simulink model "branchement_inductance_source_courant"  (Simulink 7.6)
settings: Solver=ode15s  StartTime=0.0  StopTime=0.015  RelTol=1e-3
StopFcn:
  | close all
  | load VI.mat
  | plotyy(x(1,:),x(2,:),x(1,:),x(3,:))
  | grid
  | title('Tension et courant dans le circuit LC')
  | xlabel('temps')
libraries: powerlib x8

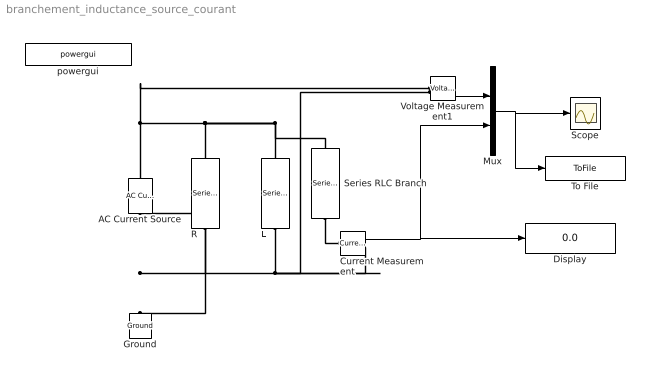
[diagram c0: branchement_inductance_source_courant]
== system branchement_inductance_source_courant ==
  AC Current Source : powerlib/Electrical Sources/AC Current Source  DialogController=POWERSYS.PowerSysDialog  SystemSampleTime=-1  Amplitude=10  Phase=0  Frequency=60  SampleTime=0  Measurements=None
  Current Measurement : powerlib/Measurements/Current Measurement  DialogController=POWERSYS.PowerSysDialog  SystemSampleTime=-1  PhasorSimulation=off  OutputType=Complex  PSBequivalent=0
  Display : Display
  Ground : powerlib/Elements/Ground  DialogController=POWERSYS.PowerSysDialog  PhysicalDomain=powersysdomain  SubClassName=unknown  LeftPortType=p1  RightPortType=p1  LConnTagsString=a
  L : powerlib/Elements/Series RLC Branch  DialogController=POWERSYS.PowerSysDialog  PhysicalDomain=powersysdomain  SubClassName=unknown  LeftPortType=p1  RightPortType=p1  LConnTagsString=__new0  RConnTagsString=__new0  BranchType=L  Resistance=1  Inductance=1e-3  SetiL0=off  InitialCurrent=0  Capacitance=1e-6  Setx0=off  InitialVoltage=0  Measurements=None
  Mux : Mux  Inputs=2
  R : powerlib/Elements/Series RLC Branch  DialogController=POWERSYS.PowerSysDialog  PhysicalDomain=powersysdomain  SubClassName=unknown  LeftPortType=p1  RightPortType=p1  LConnTagsString=__new0  RConnTagsString=__new0  BranchType=R  Resistance=1e6  Inductance=1e-3  SetiL0=off  InitialCurrent=0  Capacitance=1e-6  Setx0=off  InitialVoltage=0  Measurements=None
  Scope : Scope
  Series RLC Branch : powerlib/Elements/Series RLC Branch  DialogController=POWERSYS.PowerSysDialog  PhysicalDomain=powersysdomain  SubClassName=unknown  LeftPortType=p1  RightPortType=p1  LConnTagsString=__new0  RConnTagsString=__new0  BranchType=RL  Resistance=1  Inductance=1e-3  SetiL0=off  InitialCurrent=0  Capacitance=1e-6  Setx0=off  InitialVoltage=0  Measurements=None
  To File : ToFile  Filename=VI.mat  MatrixName=x
  Voltage Measurement1 : powerlib/Measurements/Voltage Measurement  DialogController=POWERSYS.PowerSysDialog  SystemSampleTime=-1  PhasorSimulation=off  OutputType=Complex  PSBequivalent=0
  powergui : powerlib/powergui  Priority=1  SystemSampleTime=-1  SimulationMode=Continuous  SampleTime=50e-6  frequency=60  SPID=off  DisableSnubberDevices=off  DisableRonSwitches=off  DisableVfSwitches=off  SwTol=0  Interpol=off  frequencyindice=60  echomessages=off  HookPort=off  DisplayEquations=off  FunctionMessages=off  EnableUseOfTLC=off  x0status=blocks  RestoreLinks=warning  ResistiveCurrentMeasurement=off  Ylog=off  Xlog=on  ShowGrid=off  save=off  variable=ZData  ZoomFFT=off  StartTime=0.0  cycles=1  DisplayStyle=1  fundamental=60  FreqAxis=off  MaxFrequency=1000  frequencyindicesteady=1  display=off  methode=off
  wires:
  Voltage Measurement1/1 -> Mux/1
  Mux/1 -> Scope/1, To File/1
  Current Measurement/1 -> Mux/2, Display/1
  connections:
  Ground/LConn1 -- AC Current Source/LConn1 -- L/LConn1 -- Current Measurement/RConn1 -- Voltage Measurement1/LConn2 -- R/LConn1
  L/RConn1 -- Series RLC Branch/RConn1 -- AC Current Source/RConn1 -- Voltage Measurement1/LConn1 -- R/RConn1
  Series RLC Branch/LConn1 -- Current Measurement/LConn1
